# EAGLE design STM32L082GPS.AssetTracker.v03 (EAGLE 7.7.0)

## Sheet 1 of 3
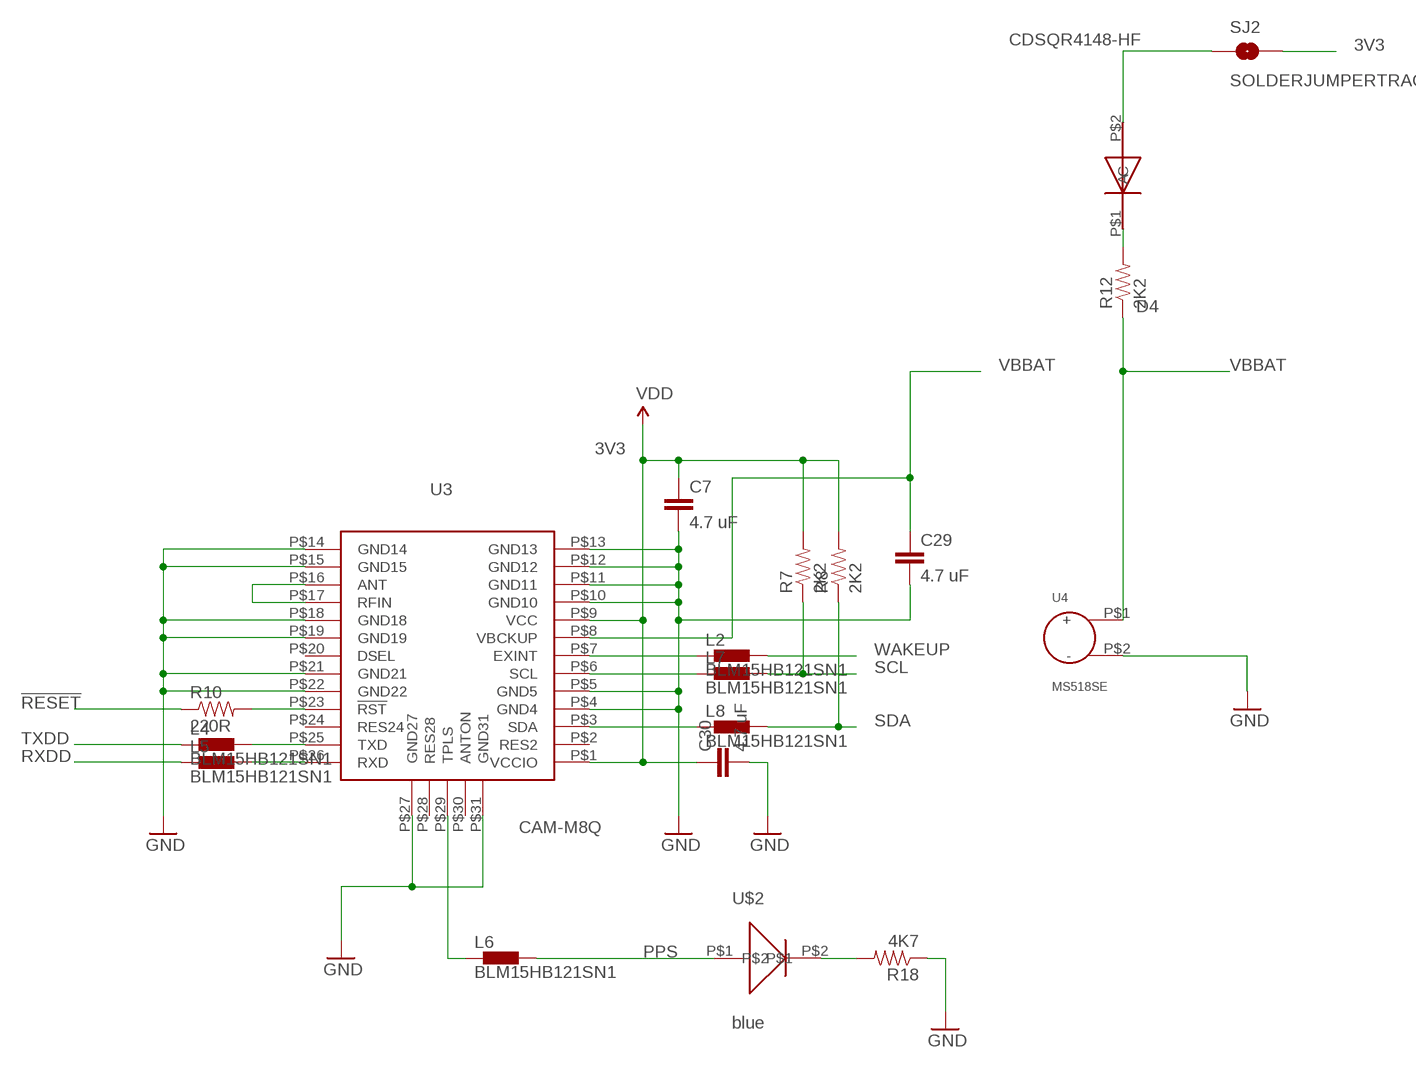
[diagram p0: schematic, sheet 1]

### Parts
C7  4.7 uF  0402CAP.KW  [0402-CAP]
C29  4.7 uF  0402CAP.KW  [0402-CAP]
C30  4.7 uF  0402CAP.KW  [0402-CAP]
D4  CDSQR4148-HF  [CDSQR4148-HF]
L2  BLM15HB121SN1  [0402]
L4  BLM15HB121SN1  [0402]
L5  BLM15HB121SN1  [0402]
L6  BLM15HB121SN1  [0402]
L7  BLM15HB121SN1  [0402]
L8  BLM15HB121SN1  [0402]
R7  2K2  0402RES.KW  [0402-RES]
R8  2K2  0402RES.KW  [0402-RES]
R10  220R  0402RES.KW  [0402-RES]
R12  2K2  0402RES.KW  [0402-RES]
R18  4K7  0402RES.KW  [0402-RES]
SJ2  SOLDERJUMPERTRACE  [SJ_2S-TRACE]
U3  CAM-M8Q  [CAM-M8Q]
U4  MS518SE  [MS518SE]
U$2  blue  0402LED  [0402LED]

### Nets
3V3: C7.1 C30.1 R7.2 R8.2 SJ2.2 U3.P$1(VCCIO) U3.P$9(VCC) ; supply symbol labelled VDD ; also sheet 2,3
!RESET: R10.1
GND: C7.2 C29.2 C30.2 R18.1 U3.P$4(GND4) U3.P$5(GND5) U3.P$10(GND10) U3.P$11(GND11) U3.P$12(GND12) U3.P$13(GND13) U3.P$14(GND14) U3.P$15(GND15) U3.P$18(GND18) U3.P$19(GND19) U3.P$21(GND21) U3.P$22(GND22) U3.P$27(GND27) U3.P$31(GND31) U4.P$2(-) ; also sheet 2,3
N$4: D4.P$2(A) SJ2.1
N$5: D4.P$1(C) R12.2
N$6: L2.1 U3.P$7(EXINT)
N$8: R18.2 U$2.P$2
N$10: L7.1 U3.P$6(SCL)
N$23: L8.1 U3.P$3(SDA)
N$43: L4.2 U3.P$25(TXD)
N$44: L5.2 U3.P$26(RXD)
N$45: U3.P$16(ANT) U3.P$17(RFIN)
N$46: R10.2 U3.P$23(!RST)
N$47: L6.1 U3.P$29(TPLS)
PPS: L6.2 U$2.P$1 ; also sheet 3
RXDD: L5.1 ; also sheet 3
SCL: L7.2 R7.1 ; also sheet 2,3
SDA: L8.2 R8.1 ; also sheet 2,3
TXDD: L4.1 ; also sheet 3
VBBAT: C29.1 R12.1 U3.P$8(VBCKUP) U4.P$1(+)
WAKEUP: L2.2 ; also sheet 3
Unconnected: U3.P$2(RES2) U3.P$20(DSEL) U3.P$24(RES24) U3.P$28(RES28) U3.P$30(ANTON)

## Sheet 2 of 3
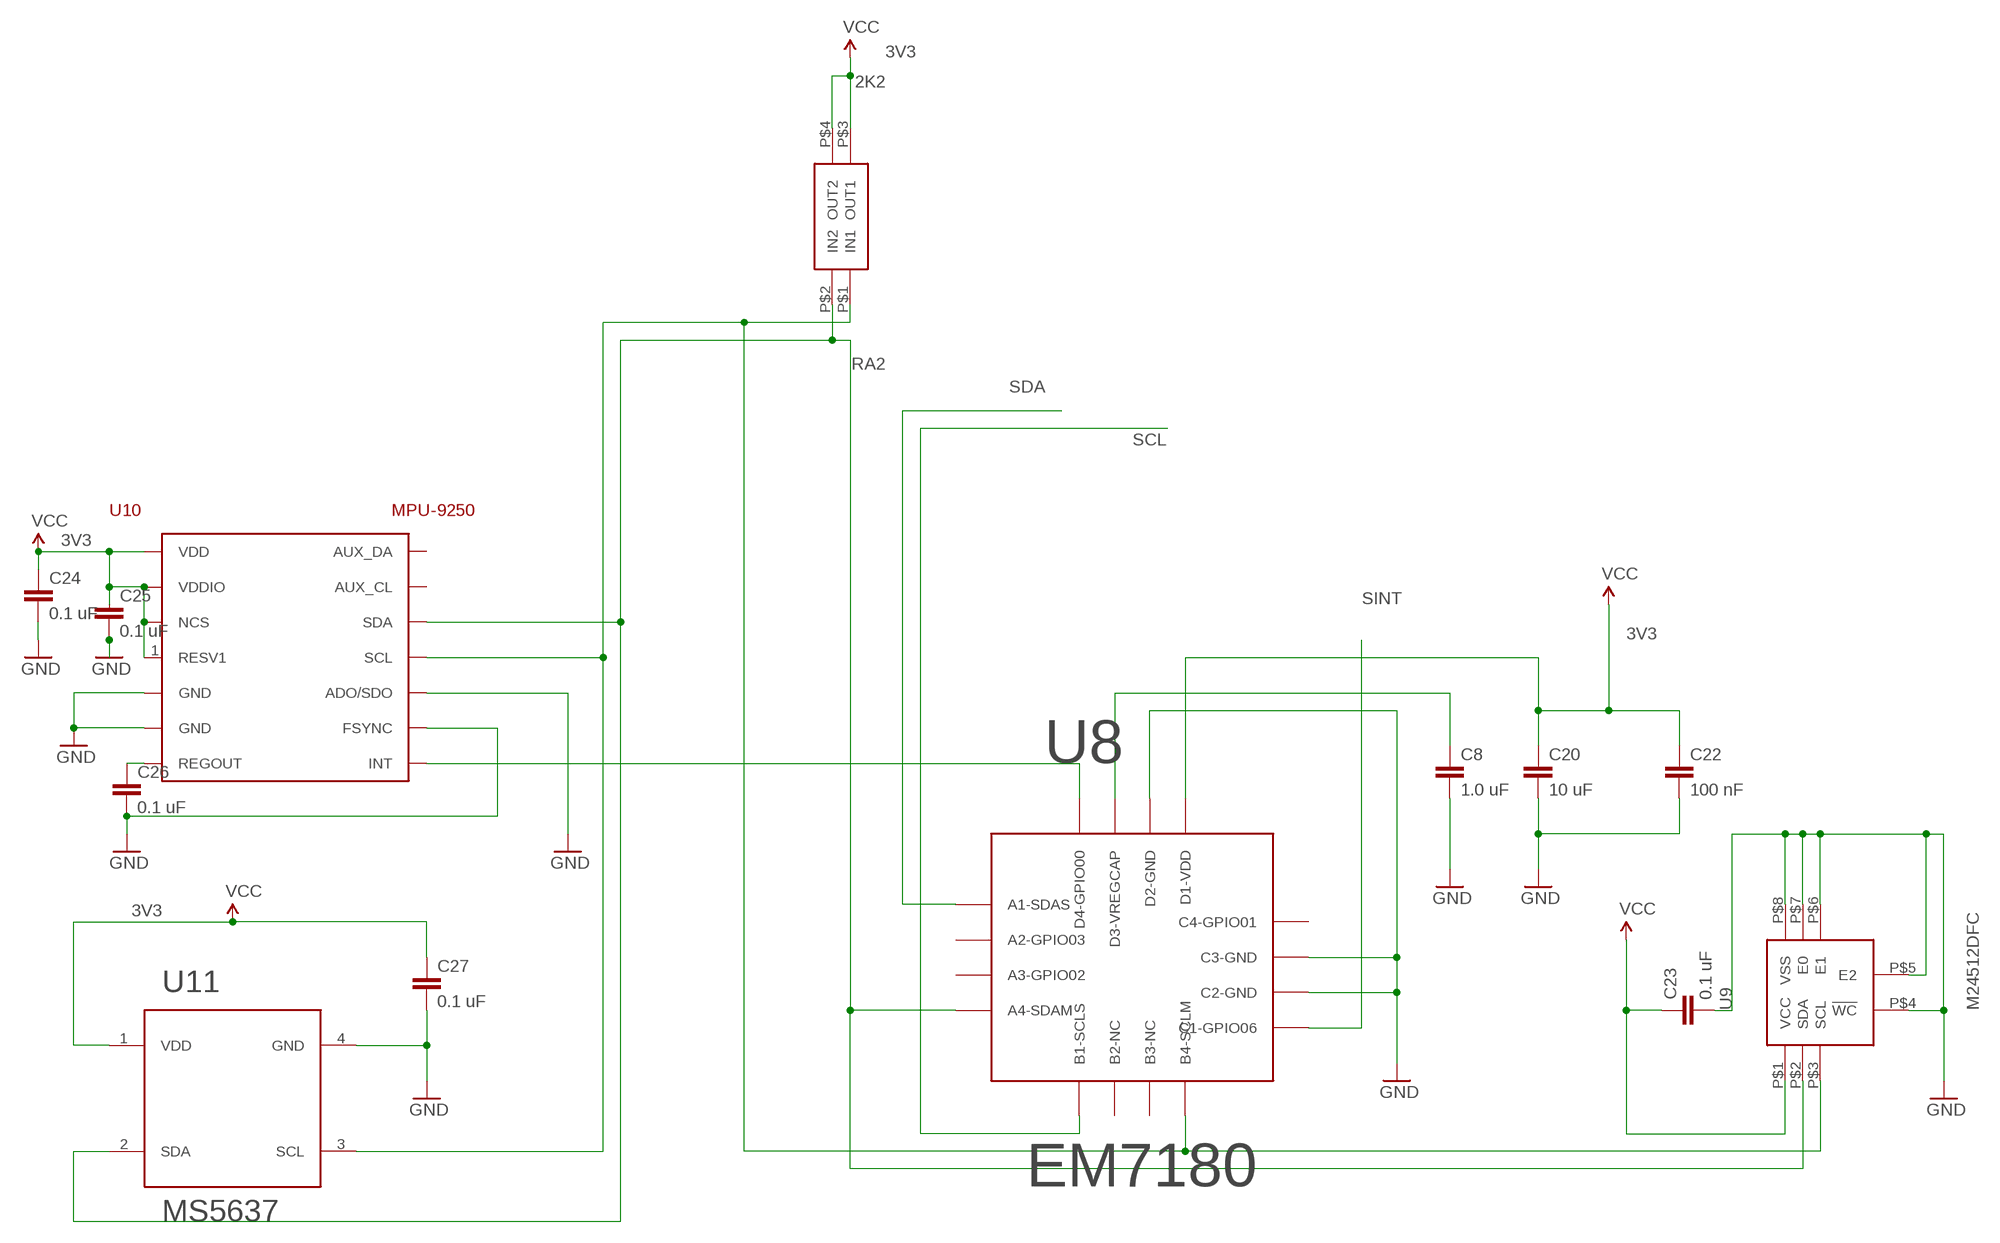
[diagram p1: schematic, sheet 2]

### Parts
C8  1.0 uF  CAP0402-CAP  [0402-CAP]
C20  10 uF  CAP0402-CAP  [0402-CAP]
C22  100 nF  CAP0402-CAP  [0402-CAP]
C23  0.1 uF  CAP0402-CAP  [0402-CAP]
C24  0.1 uF  CAP0402-CAP  [0402-CAP]
C25  0.1 uF  CAP0402-CAP  [0402-CAP]
C26  0.1 uF  CAP0402-CAP  [0402-CAP]
C27  0.1 uF  CAP0402-CAP  [0402-CAP]
RA2  2K2  EXB24V  [EXB24V]
U8  EM7180  [WL-CSP16]
U9  M24512DFC  [M24512DFC]
U10  MPU-9250  [MPU-9250]
U11  MS5637  [MS5637QFN-4]

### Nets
3V3: C20.1 C22.1 C23.1 C24.1 C25.1 C27.1 RA2.P$3(OUT1) RA2.P$4(OUT2) U8.P$13(D1-VDD) U9.P$1(VCC) U10.1(RESV1) U10.8(VDDIO) U10.13(VDD) U10.22(NCS) U11.1(VDD) ; supply symbol labelled VCC ; also sheet 1,3
GND: C8.2 C20.2 C22.2 C23.2 C24.2 C25.2 C26.2 C27.2 U8.P$10(C2-GND) U8.P$11(C3-GND) U8.P$14(D2-GND) U9.P$4(!WC) U9.P$5(E2) U9.P$6(E1) U9.P$7(E0) U9.P$8(VSS) U10.9(ADO/SDO) U10.11(FSYNC) U10.18(GND) U10.20(GND) U11.4(GND) ; also sheet 1,3
N$19: U8.P$16(D4-GPIO00) U10.12(INT)
N$26: C8.1 U8.P$15(D3-VREGCAP)
N$40: C26.1 U10.10(REGOUT)
SCL: U8.P$5(B1-SCLS) ; also sheet 1,3
SCL2: RA2.P$1(IN1) U8.P$8(B4-SCLM) U9.P$3(SCL) U10.23(SCL) U11.3(SCL)
SDA: U8.P$1(A1-SDAS) ; also sheet 1,3
SDA2: RA2.P$2(IN2) U8.P$4(A4-SDAM) U9.P$2(SDA) U10.24(SDA) U11.2(SDA)
SINT: U8.P$9(C1-GPIO06) ; also sheet 3
Unconnected: U8.P$2(A2-GPIO03) U8.P$3(A3-GPIO02) U8.P$6(B2-NC) U8.P$7(B3-NC) U8.P$12(C4-GPIO01) U10.7(AUX_CL) U10.21(AUX_DA)

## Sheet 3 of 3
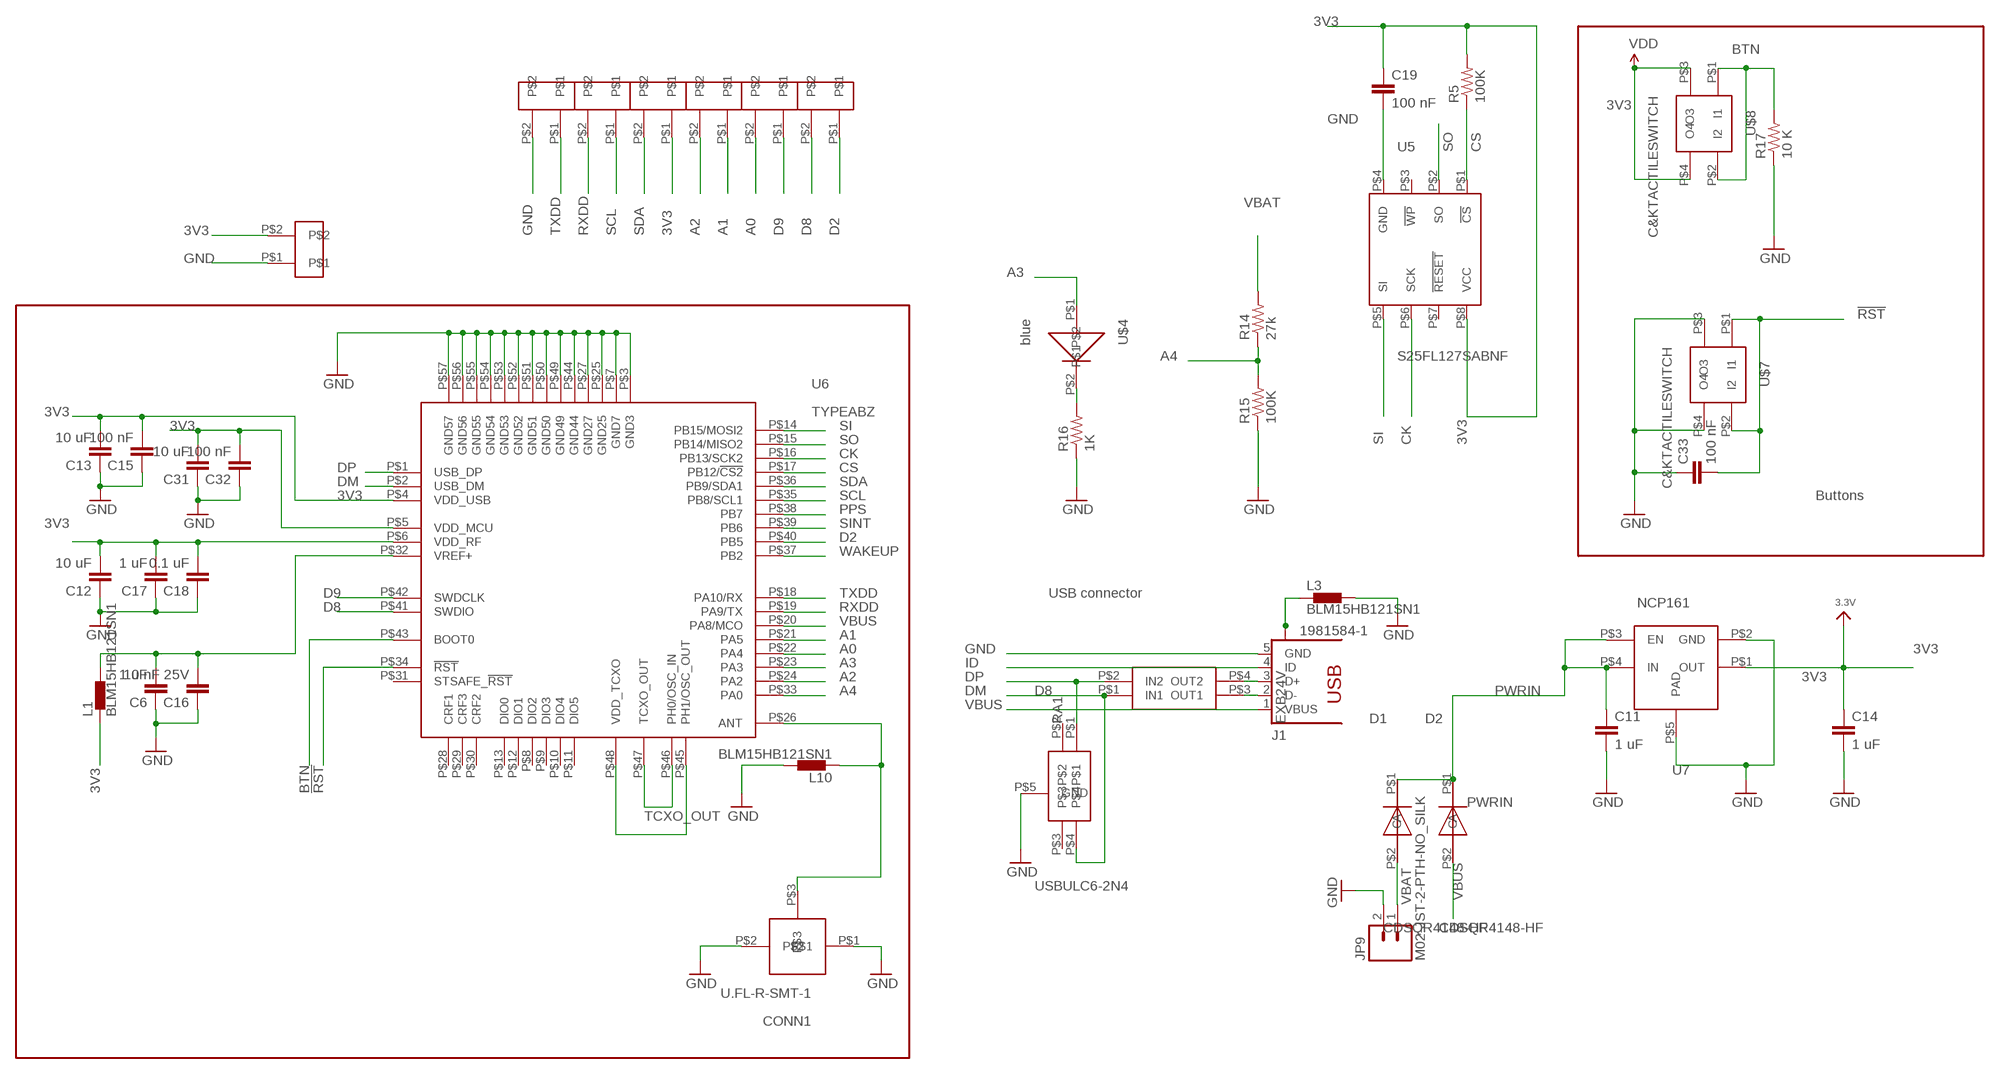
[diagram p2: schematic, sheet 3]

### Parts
C6  1 uF  0402CAP.KW  [0402-CAP]
C11  1 uF  CAP0402-CAP  [0402-CAP]
C12  10 uF  0402CAP.KW  [0402-CAP]
C13  10 uF  0402CAP.KW  [0402-CAP]
C14  1 uF  CAP0402-CAP  [0402-CAP]
C15  100 nF  0402CAP.KW  [0402-CAP]
C16  10 nF 25V  0402CAP.KW  [0402-CAP]
C17  1 uF  0402CAP.KW  [0402-CAP]
C18  0.1 uF  0402CAP.KW  [0402-CAP]
C19  100 nF  0402CAP.KW  [0402-CAP]
C31  10 uF  0402CAP.KW  [0402-CAP]
C32  100 nF  0402CAP.KW  [0402-CAP]
C33  100 nF  0402CAP.KW  [0402-CAP]
CONN1  U.FL-R-SMT-1  [U.FL-R-SMT-1]
D1  CDSQR4148-HF  [CDSQR4148-HF]
D2  CDSQR4148-HF  [CDSQR4148-HF]
D8  USBULC6-2N4  [USBULC6-2N4]
J1  1981584-1  [1981584-1]
JP9  M02-JST-2-PTH-NO_SILK  [JST-2-PTH-NS]
L1  BLM15HB121SN1  [0402]
L3  BLM15HB121SN1  [0402]
L10  BLM15HB121SN1  [0402]
R5  100K  0402RES.KW  [0402-RES]
R14  27k  0402RES.KW  [0402-RES]
R15  100K  0402RES.KW  [0402-RES]
R16  1K  0402RES.KW  [0402-RES]
R17  10 K  0402RES.KW  [0402-RES]
RA1  EXB24V  [EXB24V]
U5  S25FL127SABNF  [WSON-8]
U6  TYPEABZ  [TYPEABZ]
U7  NCP161  [NCP161]
U$4  blue  0402LED  [0402LED]
U$7  C&KTACTILESWITCH  [C&KTACTILESWITCH]
U$8  C&KTACTILESWITCH  [C&KTACTILESWITCH]
U$11  HN02  [HN02]
U$12  HN02  [HN02]
U$13  HN02  [HN02]
U$14  HN02  [HN02]
U$16  HN02  [HN02]
U$17  HN02  [HN02]
U$36  HN02  [HN02]

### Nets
3V3: C12.2 C13.2 C14.1 C15.2 C17.2 C18.2 C19.1 C31.2 C32.2 L1.1 R5.2 U5.P$8(VCC) U6.P$4(VDD_USB) U6.P$5(VDD_MCU) U6.P$6(VDD_RF) U7.P$1(OUT) U$8.P$3(O3) U$8.P$4(O4) U$13.P$1 U$36.P$2 ; supply symbol labelled VDD, 3.3V ; also sheet 1,2
!RST: C33.2 U6.P$34(!RST) U$7.P$1(I1) U$7.P$2(I2)
A0: U6.P$22(PA4) U$17.P$2
A1: U6.P$21(PA5) U$14.P$1
A2: U6.P$24(PA2) U$14.P$2
A3: U6.P$23(PA3) U$4.P$1
A4: R14.1 R15.2 U6.P$33(PA0)
AREF: C6.2 C16.2 L1.2 U6.P$32(VREF+)
BTN: R17.2 U6.P$43(BOOT0) U$8.P$1(I1) U$8.P$2(I2)
CK: U5.P$6(SCK) U6.P$16(PB13/SCK2)
CS: R5.1 U5.P$1(!CS) U6.P$17(PB12/!CS2)
D2: U6.P$40(PB5) U$16.P$1
D8: U6.P$41(SWDIO) U$16.P$2
D9: U6.P$42(SWDCLK) U$17.P$1
DM: D8.P$4 RA1.P$1(IN1) U6.P$2(USB_DM)
DP: D8.P$1 RA1.P$2(IN2) U6.P$1(USB_DP)
GND: C6.1 C11.2 C12.1 C13.1 C14.2 C15.1 C16.1 C17.1 C18.1 C19.2 C31.1 C32.1 C33.1 CONN1.P$1 CONN1.P$2 D8.P$5(GND) J1.5(GND) JP9.2 L3.2 L10.2 R15.1 R16.1 R17.1 U5.P$4(GND) U6.P$3(GND3) U6.P$7(GND7) U6.P$25(GND25) U6.P$27(GND27) U6.P$44(GND44) U6.P$49(GND49) U6.P$50(GND50) U6.P$51(GND51) U6.P$52(GND52) U6.P$53(GND53) U6.P$54(GND54) U6.P$55(GND55) U6.P$56(GND56) U6.P$57(GND57) U7.P$2(GND) U7.P$5(PAD) U$7.P$3(O3) U$7.P$4(O4) U$11.P$2 U$36.P$1 ; also sheet 1,2
ID: J1.4(ID)
N$7: U6.P$45(PH1/OSC_OUT) U6.P$48(VDD_TCXO)
N$11: R16.2 U$4.P$2
N$31: J1.3(D+) RA1.P$4(OUT2)
N$32: CONN1.P$3 L10.1 U6.P$26(ANT)
N$33: J1.2(D-) RA1.P$3(OUT1)
PPS: U6.P$38(PB7) ; also sheet 1
PWRIN: C11.1 D1.P$1(C) D2.P$1(C) U7.P$3(EN) U7.P$4(IN)
RXDD: U6.P$19(PA9/TX) U$12.P$2 ; also sheet 1
SCL: U6.P$35(PB8/SCL1) U$12.P$1 ; also sheet 1,2
SDA: U6.P$36(PB9/SDA1) U$13.P$2 ; also sheet 1,2
SI: U5.P$5(SI) U6.P$14(PB15/MOSI2)
SINT: U6.P$39(PB6) ; also sheet 2
SO: U5.P$2(SO) U6.P$15(PB14/MISO2)
TCXO_OUT: U6.P$46(PH0/OSC_IN) U6.P$47(TCXO_OUT)
TXDD: U6.P$18(PA10/RX) U$11.P$1 ; also sheet 1
USB_SHIELD1: J1.S1 J1.S2 J1.S3 J1.S4 L3.1
VBAT: D1.P$2(A) JP9.1 R14.2
VBUS: D2.P$2(A) J1.1(VBUS) U6.P$20(PA8/MCO)
WAKEUP: U6.P$37(PB2) ; also sheet 1
Unconnected: D8.P$2 D8.P$3 U5.P$3(!WP) U5.P$7(!RESET) U6.P$8(DIO2) U6.P$9(DIO3) U6.P$10(DIO4) U6.P$11(DIO5) U6.P$12(DIO1) U6.P$13(DIO0) U6.P$28(CRF1) U6.P$29(CRF3) U6.P$30(CRF2) U6.P$31(STSAFE_!RST)

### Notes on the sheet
- Buttons
- USB connector

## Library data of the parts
C6 C7 C12 C13 C15-C19 C29-C33 = SparkFun-Capacitors:0402CAP.KW
C8 C11 C14 C20 C22-C27 = SparkFun-Capacitors:CAP: Capacitor
CONN1 = Kris:U.FL-R-SMT-1: U.FL-R-SMT-1
D1 D2 D4 = Kris:CDSQR4148-HF: ComChip's CDSQR4148-HF high speed 150 mA Io diode
D8 = Kris:USBULC6-2N4: ST TVS diode ESD Protection USBULC6-2N4
J1 = con-usb:1981584-1: Receptacle, micro-USB, type A/B Tyco Electronics; MF: Hirose; MPN: ZX62-AB-5PA(11)
JP9 = SparkFun-Connectors:M02: Standard 2-pin 0.1" header. Use with
L1-L8 L10 = inductors:BLM15H: EMIFIL (R) Chip Ferrite Bead for GHz Noise
R5 R7 R8 R10 R12 R14-R18 = SparkFun-Resistors:0402RES.KW
RA1 RA2 = Kris:EXB24V: Panasonic EXB24 22 Ohm series resistor pair
SJ2 = SparkFun-Passives:SOLDERJUMPER: Solder Jumper
U3 = ubloxLib:CAM-M8Q: CAM-M8Q GPS/GNSS Module https://www.u-blox.com/sites/default/files/CAM-M8_HardwareIntegrationManual_%28UBX-14000014%29.pdf
U4 = Kris:MS518SE: S518SE 3 V rechargable Li battery
U5 = Kris:S25FL127SABNF: S225FL127SABNF1101 128 Mbit Spansion flash in WSON-8 package
U6 = Kris:TYPEABZ: CMWX1ZZABZ-078
U7 = Kris:NCP161: NCP161 3V3 LDO voltage regulator
U8 = SparkFun-DigitalIC:EM7180: WL-CSP19 package for the EM7180 SENtral sensor fusion hub
U9 = Kris:M24512DFC: ST's M24512DFC6 512 Mbit EEPROM
U10 = SparkFun-Sensors:MPU-9250: The MPU-9250 is a 9-axis motion sensor that contains an accelerometer/gyro sensor (MPU-6500) combined with a magnetometer (AK8963).
U11 = SparkFun-DiscreteSemi:MS5637: MS5637 I2C pressure sensor in QFN-4 package by Measurement Specialties
U$2 U$4 = Kris:0402LED: 0402led
U$7 U$8 = Kris:C&KTACTILESWITCH: C&K Tactile Switch 611-PTS810SJS250SMTR
U$11-U$14 U$16 U$17 U$36 = Kris:HN02: 0.1 inch header

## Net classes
1 USB: width 0.254 mm, drill 0.33 mm, clearance 0.159 mm
2 Top GND Pour: clearance 0.762 mm to class 1

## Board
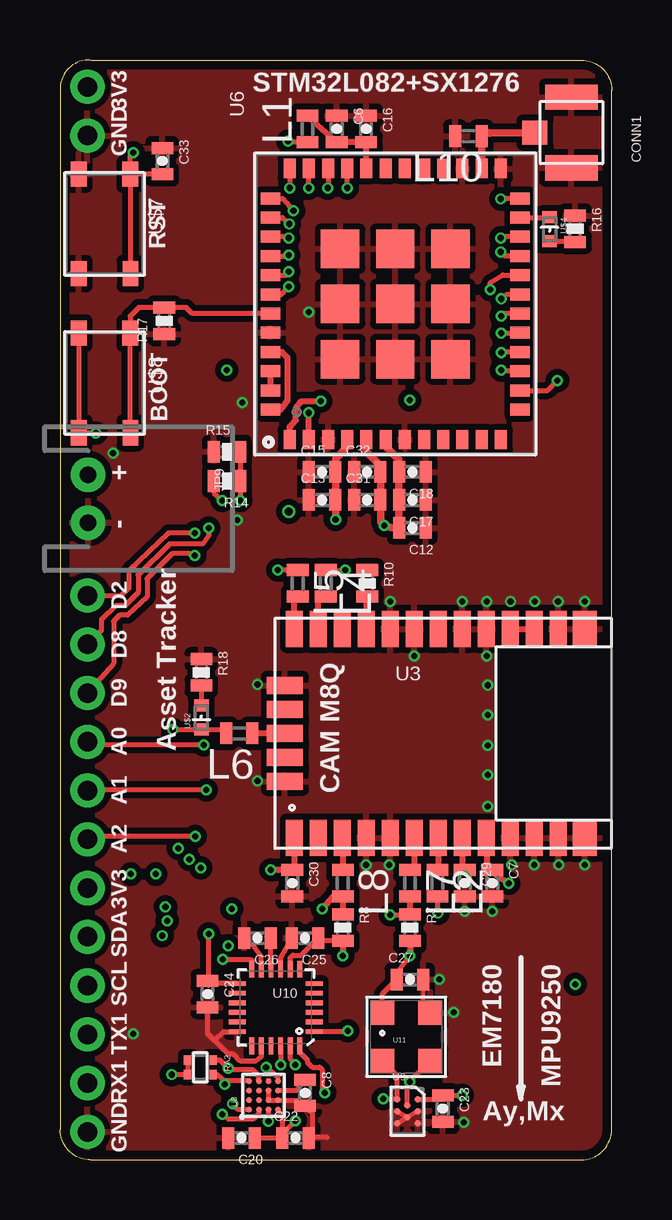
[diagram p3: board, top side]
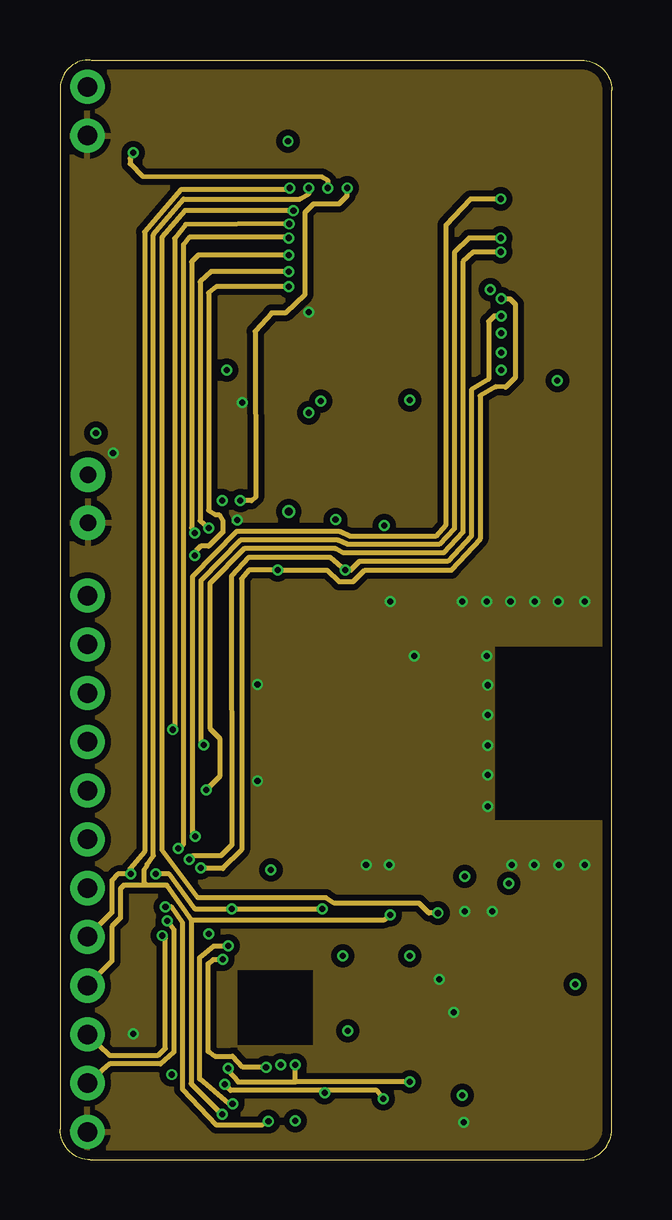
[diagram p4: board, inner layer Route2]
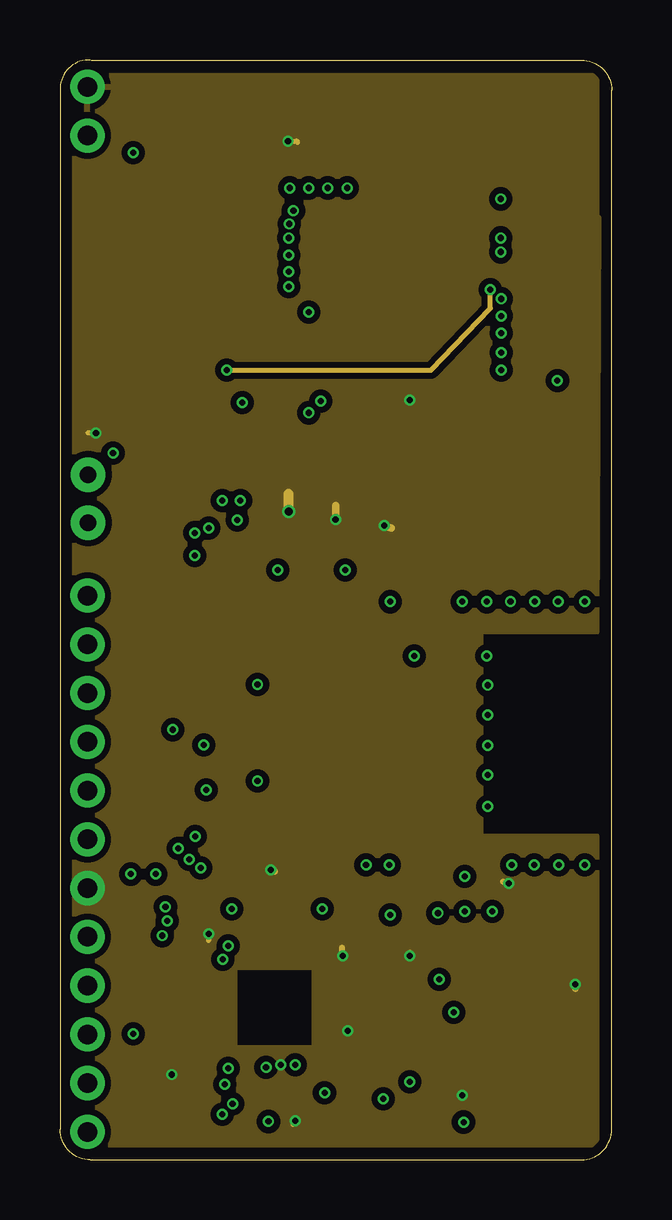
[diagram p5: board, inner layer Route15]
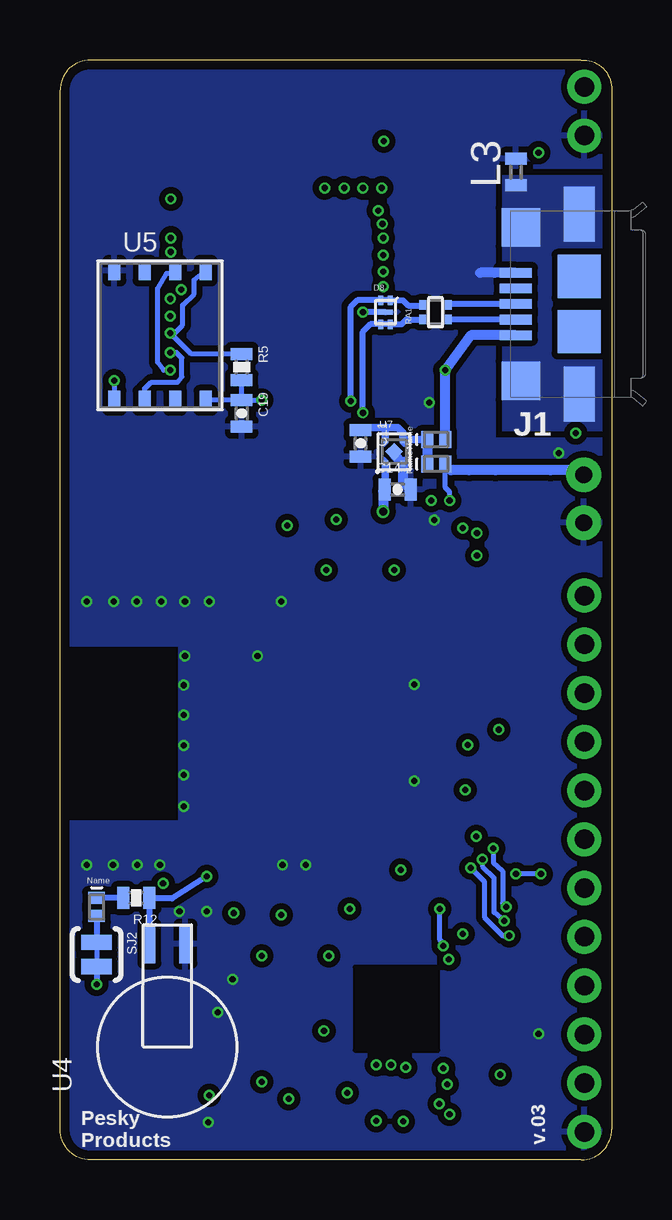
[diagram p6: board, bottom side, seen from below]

Size 22.99 x 45.85 mm. Coordinates in mm from the lower left corner, seen from the top.
Outline: 1.27,45.85 arc90 0,44.7 0,1.27 arc90 1.27,0 21.72,0 arc90 22.99,1.27 22.99,44.58 arc90 21.72,45.85 1.29,45.85
Copper layers (1*2*15*16): Top 0.035559375mm / dielectric 0.17018125mm / Route2 0.01778125mm / dielectric 47mil / Route15 0.01778125mm / dielectric 0.17018125mm / Bottom 0.035559375mm
Design rules "OSHPark-4layer *": minimum track width 5mil, minimum drill 10mil, track to track 5mil, track to pad 5mil, pad to pad 5mil, via to via 5mil, smd to smd 5mil, copper to edge 15mil, drill to drill 6mil, minimum pad ring 4mil, minimum via ring 4mil, stop-mask expansion 4mil, vias tented up to drill 20mil, thermal gap 10mil

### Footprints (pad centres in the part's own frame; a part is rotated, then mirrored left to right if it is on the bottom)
0402-CAP = smd 0.5 x 0.9: 1 -0.55,0; 2 0.55,0
U.FL-R-SMT-1 = smd 1.05 x 2.2: P$1 -1.475,0; P$2 1.475,0 | smd 1 x 1.05: P$3 0,-1.525
CDSQR4148-HF = smd 0.7 x 0.5: P$1 0,0.375; P$2 0,-0.375
USBULC6-2N4 = smd 0.2 x 0.4: P$1 0.2,0.5; P$2 -0.2,0.5; P$3 -0.2,-0.5; P$4 0.2,-0.5 | smd 0.6 x 0.2: P$5 0,0
1981584-1 = smd 0.4 x 1.35: 1 -1.3,4.1; 2 -0.65,4.1; 3 0,4.1; 4 0.65,4.1; 5 1.3,4.1 | smd 1.8 x 1.8: M1 -1.15,1.45; M2 1.15,1.45 | smd 2.3 x 1.3: S1 -3.75,1.45; S2 3.75,1.45 | smd 1.6 x 1.6: S3 -3.2,3.885; S4 3.2,3.885
JST-2-PTH-NS = drill 0.7 pad 1.448: 1 -1,0; 2 1,0
0402 = smd 0.5 x 0.9: 1 -0.55,0; 2 0.55,0
0402-RES = smd 0.5 x 0.9: 1 -0.55,0; 2 0.55,0
EXB24V = smd 0.4 x 0.36: P$1 -0.3,0.5; P$2 0.3,0.5; P$3 -0.3,-0.5; P$4 0.3,-0.5
SJ_2S-TRACE = smd 0.635 x 1.27: 1 -0.508,0; 2 0.508,0
CAM-M8Q = smd 0.7 x 1.5: P$1 0.8,0.45; P$2 1.8,0.45; P$3 2.8,0.45; P$4 3.8,0.45; P$5 4.8,0.45; P$6 5.8,0.45; P$7 6.8,0.45; P$8 7.8,0.45; P$9 8.8,0.45; P$10 9.8,0.45; P$11 10.8,0.45; P$12 11.8,0.45; P$15 11.8,9.15; P$16 10.8,9.15; P$17 9.8,9.15; P$18 8.8,9.15; P$19 7.8,9.15; P$20 6.8,9.15; P$21 5.8,9.15; P$22 4.8,9.15; P$23 3.8,9.15; P$24 2.8,9.15; P$25 1.8,9.15; P$26 0.8,9.15 | smd 1 x 1.5: P$13 12.9,0.45; P$14 12.9,9.15 | smd 1.5 x 0.7: P$27 0.4,6.8; P$28 0.4,5.8; P$29 0.4,4.8; P$30 0.4,3.8; P$31 0.4,2.8
MS518SE = smd 1.6 x 0.5: P$1 4.3,0.75; P$2 4.3,-0.75
WSON-8 = smd 0.5 x 0.8: P$1 1.905,2.7; P$2 0.635,2.7; P$3 -0.635,2.7; P$4 -1.905,2.7; P$5 -1.905,-2.7; P$6 -0.635,-2.7; P$7 0.635,-2.7; P$8 1.905,-2.7
TYPEABZ = smd 0.8 x 0.5: P$1 -5.65,4.4; P$2 -5.65,3.6; P$3 -5.65,2.8; P$4 -5.65,2; P$5 -5.65,1.2; P$6 -5.65,0.4; P$7 -5.65,-0.4; P$8 -5.65,-1.2; P$9 -5.65,-2; P$10 -5.65,-2.8; P$11 -5.65,-3.6; P$12 -5.65,-4.4; P$25 5.65,-4.4; P$26 5.65,-3.6; P$27 5.65,-2.8; P$28 5.65,-2; P$29 5.65,-1.2; P$30 5.65,-0.4; P$31 5.65,0.4; P$32 5.65,1.2; P$33 5.65,2; P$34 5.65,2.8; P$35 5.65,3.6; P$36 5.65,4.4 | smd 0.5 x 0.8: P$13 -4.4,-5.2; P$14 -3.6,-5.2; P$15 -2.8,-5.2; P$16 -2,-5.2; P$17 -1.2,-5.2; P$18 -0.4,-5.2; P$19 0.4,-5.2; P$20 1.2,-5.2; P$21 2,-5.2; P$22 2.8,-5.2; P$23 3.6,-5.2; P$24 4.4,-5.2; P$37 4.4,5.2; P$38 3.6,5.2; P$39 2.8,5.2; P$40 2,5.2; P$41 1.2,5.2; P$42 0.4,5.2; P$43 -0.4,5.2; P$44 -1.2,5.2; P$45 -2,5.2; P$46 -2.8,5.2; P$47 -3.6,5.2; P$48 -4.4,5.2 | smd 1.6 x 1.6: P$49 -2.3,2.3; P$50 0,2.3; P$51 2.3,2.3; P$52 -2.3,0; P$53 0,0; P$54 2.3,0; P$55 -2.3,-2.3; P$56 0,-2.3; P$57 2.3,-2.3
NCP161 = smd 0.24 x 0.24: P$1 -0.37,-0.48; P$2 0.37,-0.48; P$3 0.37,0.48; P$4 -0.37,0.48 | smd 0.52 x 0.52 rotated 45: P$5 0,0
WL-CSP16 = smd 0.24 x 0.24: P$1 -0.6,0.6; P$2 -0.2,0.6; P$3 0.2,0.6; P$4 0.6,0.6; P$5 -0.6,0.2; P$6 -0.2,0.2; P$7 0.2,0.2; P$8 0.6,0.2; P$9 -0.6,-0.2; P$10 -0.2,-0.2; P$11 0.2,-0.2; P$12 0.6,-0.2; P$13 -0.6,-0.6; P$14 -0.2,-0.6; P$15 0.2,-0.6; P$16 0.6,-0.6
M24512DFC = smd 0.27 x 0.27: P$1 0.433,0.5; P$2 -0.433,0.5; P$3 0,0.25; P$4 0.433,0; P$5 -0.433,0; P$6 0,-0.25; P$7 0.433,-0.5; P$8 -0.433,-0.5
MPU-9250 = smd 0.7 x 0.2: 1 -1.6,1; 2 -1.6,0.6; 3 -1.6,0.2; 4 -1.6,-0.2; 5 -1.6,-0.6; 6 -1.6,-1; 13 1.6,-1; 14 1.6,-0.6; 15 1.6,-0.2; 16 1.6,0.2; 17 1.6,0.6; 18 1.6,1 | smd 0.2 x 0.7: 7 -1,-1.6; 8 -0.6,-1.6; 9 -0.2,-1.6; 10 0.2,-1.6; 11 0.6,-1.6; 12 1,-1.6; 19 1,1.6; 20 0.6,1.6; 21 0.2,1.6; 22 -0.2,1.6; 23 -0.6,1.6; 24 -1,1.6
MS5637QFN-4 = smd 1 x 1: 1 -1,1; 2 -1,-1; 3 1,-1; 4 1,1
0402LED = smd 0.5 x 0.6: P$1 -0.5,0; P$2 0.5,0
C&KTACTILESWITCH = smd 1.05 x 0.65: P$1 -2.075,1.073; P$2 2.075,1.075; P$3 -2.075,-1.075; P$4 2.075,-1.075
HN02 = drill 0.813 pad 1.422: P$1 0,0; P$2 -2.032,0

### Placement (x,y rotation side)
C6  11.53,42.98 270 top
C7  18.01,11.53 270 top
C8  10.21,2.79 270 top
C11  10.46,29.87 270 bottom
C12  14.68,26.34 180 top
C13  10.92,27.51 0 top
C14  8.92,27.94 0 bottom
C15  10.92,28.68 0 top
C16  12.75,42.98 270 top
C17  14.68,27.51 180 top
C18  14.68,28.68 180 top
C19  15.42,31.11 270 bottom
C20  7.57,0.91 180 top
C22  9.8,0.91 0 top
C23  15.95,2.13 270 top
C24  6.15,6.91 270 top
C25  10.21,9.25 180 top
C26  8.23,9.25 180 top
C27  14.58,7.52 0 top
C29  16.87,11.53 270 top
C30  9.68,11.53 270 top
C31  12.8,27.51 0 top
C32  12.8,28.68 0 top
C33  4.27,41.63 270 top
CONN1  21.31,42.82 270 top
D1  7.32,29.01 90 bottom
D2  7.32,30.02 90 bottom
D4  21.46,10.54 0 bottom
D8  9.42,35.33 0 bottom
J1  -0.1,35.68 90 bottom
JP9  1.17,27.56 270 top
L1  10.31,42.98 90 top
L2  15.72,11.53 270 top
L3  3.99,41.17 90 bottom
L4  11.07,24.03 270 top
L5  9.91,24.03 270 top
L6  7.47,17.78 180 top
L7  14.58,11.53 270 top
L8  11.79,11.53 270 top
L10  17.02,42.67 180 top
R5  15.42,33.05 270 bottom
R7  14.58,9.68 270 top
R8  11.79,9.68 270 top
R10  12.8,24.03 270 top
R12  19.81,10.92 180 bottom
R14  6.96,28.3 180 top
R15  6.96,29.51 0 top
R16  21.46,38.81 270 top
R17  4.34,34.98 90 top
R18  5.89,20.32 270 top
RA1  7.34,35.33 90 bottom
RA2  5.84,3.86 270 top
SJ2  21.46,8.56 270 bottom
U3  8.97,12.98 0 top
U4  18.52,4.7 90 bottom
U5  18.82,34.37 0 bottom
U6  13.97,35.68 90 top
U7  9.07,29.51 0 bottom
U8  8.48,2.69 90 top
U9  14.48,2.03 0 top
U10  8.99,6.35 180 top
U11  14.43,5.13 0 top
U$2  5.89,18.44 90 top
U$4  20.4,38.79 270 top
U$7  1.85,39.01 270 top
U$8  1.85,32.38 270 top
U$11  1.14,3.2 90 top
U$12  1.14,7.26 90 top
U$13  1.14,11.33 90 top
U$14  1.14,15.39 90 top
U$16  1.14,23.52 90 top
U$17  1.14,19.46 90 top
U$36  1.14,42.7 270 top

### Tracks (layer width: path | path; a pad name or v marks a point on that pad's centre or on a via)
3V3  (via drill 0.25, 0.33)
  Top 0.203: U8.P$13 9.25,1.75 C22.1 | C22.1 9.2,0.97 v9.8,1.63 | U10.22 v9.2,3.96 | U11.1 13.43,6.92 C27.1 14.03,7.78 v14.58,8.51 | v16.76,2.69 16.81,2.68 C23.1 16.05,2.53 U9.P$1 | v4.65,3.56 RA2.P$4 RA2.P$3 | R8.2 10.96,9.13 C25.1 10.05,8.53 9.7,8.53 9.59,8.42 U10.8 | v6.2,9.42 6.2,7.26 C24.1 6.17,7.35 U10.13 | U10.1 11.95,5.35 v11.99,5.38 | C20.1 C22.1 | v1.5,30.3 1.19,30.31 U$8.P$4 U$8.P$3 | L1.1 9.59,42.43 v9.5,42.47
  Top 0.254: U3.P$9 17.79,12.4 C7.1 18.18,11.88 v18.69,11.53 | R7.2 14.59,8.75 v14.58,8.51 | R8.2 v11.79,8.51 | U3.P$1 9.77,12.09 C30.1 9.11,12.08 v8.79,12.09
  Top 0.305: U6.P$4 11.97,29.73 11.48,29.23 11.48,28.68 | 11.48,28.68 C15.2 | 11.48,28.68 11.48,27.52 C13.2 11.48,27.5 v11.48,26.7 | U6.P$6 13.57,29.74 14.12,29.18 C18.2 | C18.2 | C17.2 14.12,26.37 C12.2 13.78,26.36 v13.51,26.44 13.36,26.59 C31.2 | C18.2 C17.2 | C17.2 | U6.P$5 12.77,29.52 13.36,28.93 C32.2 | C32.2 | C32.2 C31.2 | C31.2
  Route15 0.203: v9.8,1.63 9.7,1.47 | v9.2,3.96 9.25,3.96 | v16.76,2.69 16.82,2.64 | v4.65,3.56 4.78,3.56 | v6.2,9.42 6.2,9.14 | v11.99,5.38 11.94,5.38 11.89,5.33 | v1.5,30.3 1.17,30.3 | v14.58,31.67 14.55,31.77 14.63,31.7 | v9.5,42.47 9.86,42.47 9.91,42.42
  Route15 0.254: 18.47,11.61 v18.69,11.53 | v14.58,8.51 14.58,8.64 | v11.79,8.51 11.76,8.84 | v8.79,12.09 8.97,12.01 8.91,12.06 8.91,12.09 8.87,12.14 | v21.46,7.32 21.46,7.14 21.49,7.11
  Route15 0.305: v11.48,26.7 11.48,27.28 | v13.51,26.44 13.79,26.34
  Route15 0.406: v9.53,27.03 9.53,27.76
  Bottom 0.203: C19.1 U5.P$8 | C19.1 v14.59,31.66 v14.58,31.67 | C19.1 R5.2
  Bottom 0.254: SJ2.2 v21.46,7.32
  Bottom 0.305: U7.P$1 9.44,28.4 C14.1 9.53,27.86
  Bottom 0.406: 9.53,27.86 v9.53,27.03
  pour Route15 (isolate 0.254, no thermals): 0.64,0.64 0.64,39.27 22.43,39.27 22.35,22.02 17.5,22.02 17.5,13.49 22.35,13.49 22.35,0.64 10.62,0.64 10.62,8.03 7.26,8.03 7.26,4.67 10.57,4.67 10.57,0.64
  pour Route15 (isolate 0.254): 0.64,39.27 0.64,45.19 22.35,45.19 22.35,39.27
!RST  (via drill 0.25)
  Top 0.203: C33.2 U$7.P$1 | U$7.P$1 U$7.P$2 | U6.P$34 11.17,40.66 v11.15,40.51 | U$7.P$1 2.92,41.83 v3.05,41.99
  Route2 0.203: v3.05,41.99 2.93,41.75 2.93,41.52 3.45,40.99 10.92,40.97 11.18,40.82 v11.15,40.51
A0  (via drill 0.25)
  Top 0.203: U6.P$22 18.41,38.48 v18.36,38.43 | v5.99,17.3 1.27,17.3 U$17.P$2
  Route2 0.203: v18.36,38.43 17.04,38.43 16.43,37.82 16.43,26.31 15.8,25.65 11.99,25.65 11.58,25.83 7.52,25.83 5.87,24.16 5.87,17.42 v5.99,17.3
A1  (via drill 0.25)
  Top 0.203: U6.P$21 18.53,37.68 v18.36,37.85 | v6.1,15.42 1.17,15.42 U$14.P$1
  Route2 0.203: v18.36,37.85 17.22,37.85 16.79,37.44 16.79,26.16 15.98,25.3 11.81,25.3 11.48,25.48 7.67,25.48 6.25,24.03 6.25,17.98 6.66,17.58 6.66,15.98 v6.1,15.42
A2  (via drill 0.25)
  Top 0.203: U6.P$24 18.39,40.08 v18.36,40.06 | v5.64,13.49 1.32,13.49 U$14.P$2
  Route2 0.203: v18.36,40.06 17.09,40.06 16.08,38.96 16.08,26.47 15.65,25.98 12.09,25.98 11.66,26.19 7.34,26.19 5.51,24.31 5.51,13.59 v5.64,13.49
A3
  Top 0.203: U6.P$23 20.34,39.28 U$4.P$1
A4  (via drill 0.25)
  Top 0.203: R15.2 R14.1 7.51,27.52 v7.52,27.48 | v11.96,40.51 U6.P$33
  Route2 0.203: v11.96,40.51 11.96,40.18 11.63,39.85 10.57,39.85 10.21,39.5 10.21,36.07 9.4,35.31 8.81,35.31 8.13,34.54 8.15,27.61 7.98,27.48 v7.52,27.48
AREF
  Top 0.254: U6.P$32 12.77,42.41 | C16.2 C6.2 L1.2
  Top 0.305: 12.77,42.41 C16.2
BTN
  Top 0.203: U6.P$43 5.52,35.28 5.26,35.53 4.35,35.53 | 4.35,35.53 R17.2 | U$8.P$2 U$8.P$1 2.92,35.18 3.28,35.53 4.35,35.53
CK  (via drill 0.25)
  Top 0.203: U6.P$16 18.41,33.68 v18.39,33.66
  Bottom 0.203: U5.P$6 19.46,32.16 19.18,32.41 18.09,32.41 17.91,32.64 17.91,33.43 18.14,33.66 v18.39,33.66
CS  (via drill 0.25)
  Top 0.203: v18.39,34.47 19.16,34.47 U6.P$17
  Bottom 0.203: 16.9,37.05 U5.P$1 17.4,36.69 17.4,36.09 17.88,35.64 17.88,34.8 18.21,34.47 v18.39,34.47 17.52,33.59 R5.1
D2  (via drill 0.25)
  Top 0.203: U6.P$40 9.43,37.68 v9.53,37.72 | v5.61,26.14 4.52,26.14 2.87,24.54 2.87,23.82 2.54,23.5 1.17,23.5 U$16.P$1
  Route2 0.203: v9.53,37.72 5.77,37.72 5.49,37.44 5.49,26.34 v5.61,26.14
D8  (via drill 0.25)
  Top 0.203: U6.P$41 9.42,36.88 v9.53,37.03 | v6.2,26.34 6.2,26.04 5.94,25.68 4.57,25.68 3.25,24.38 3.25,23.65 2.72,23.11 2.34,23.11 1.73,22.5 1.73,22.07 U$16.P$2
  Route2 0.203: v9.53,37.03 6.3,37.03 5.84,36.6 5.84,26.64 v6.2,26.34
D9  (via drill 0.25)
  Top 0.203: U6.P$42 9.23,36.08 v9.53,36.4 | v5.61,25.2 5.61,25.25 5.39,25.27 4.67,25.27 3.63,24.23 3.63,23.47 2.82,22.71 2.49,22.71 2.24,22.45 2.24,20.7 U$17.P$1
  Route2 0.203: v9.53,36.4 6.5,36.4 6.2,36.14 6.2,27.08 6.48,26.9 6.63,26.9 6.78,26.64 6.78,26.16 6.2,25.58 5.87,25.58 5.66,25.38 v5.61,25.2
DM  (via drill 0.25)
  Top 0.254: U6.P$2 10.37,31.17 v10.36,31.14
  Bottom 0.254: v10.36,31.14 10.36,34.52 10.05,34.83 D8.P$4 8.75,34.83 8.56,35.03 RA1.P$1
DP  (via drill 0.25)
  Top 0.254: U6.P$1 9.57,30.55 9.83,30.84 9.83,31.34 10.06,31.62 v10.87,31.62
  Bottom 0.254: v10.87,31.62 10.87,35.56 10.6,35.83 D8.P$1 8.7,35.83 8.48,35.61 7.86,35.61 RA1.P$2
GND  (via drill 0.25)
  Top 0.152: C27.2 15.13,6.43 U11.4
  Top 0.203: U8.P$11 U8.P$10 U8.P$14 9.96,2.49 C8.2 10.52,1.93 10.52,1.08 C22.2 10.35,0.94 11.12,0.94 | U10.11 8.39,8.47 8.08,8.89 C26.2 | U10.9 9.19,8.42 C25.2 | U10.18 7.37,5.32 6.8,5.32 6.45,4.98 | U9.P$5 U9.P$6 | U9.P$8 U9.P$6 | U9.P$4 U9.P$6 | U10.20 8.39,4.3 8.15,4.12 7.52,4.12 7.21,4.42 7.01,4.42 6.45,4.98 | 6.45,4.98 6.43,4.98 6.15,5.26 C24.2 | 10.36,0.84 10.36,0.86
  Top 0.254: C22.2 10.35,0.87 10.36,0.86 | v10.36,35.33 10.31,35.28
  Bottom 0.254: D8.P$5 v10.36,35.33
  Bottom 0.406: J1.5 4.88,36.98 5.49,36.98 | C14.2 8.7,28.27 U7.P$2 9.07,29.41 U7.P$5
  other vias: 20.75,23.27 21.87,23.27 17.78,21.01 16.76,23.27 18.82,12.29 19.76,12.29 20.78,12.29 21.87,12.29 14.76,21.01 13.77,23.27 13.72,12.29 12.75,12.29 8.23,19.81 8.23,15.8 17.83,19.79 17.83,18.54 17.83,17.27 17.83,16.05 17.83,14.73 18.01,10.36 16.41,6.15 15.8,7.52 16.81,1.57 3.05,5.26 7.39,26.67 17.78,23.27 18.77,23.27 16.87,10.36 19.79,23.27 7.59,31.57 2.21,29.46
  pour Top (isolate 0.254): 0,0 0,39.29 22.99,39.29 23.06,21.51 17.98,21.51 17.98,14.05 22.96,14.05 22.96,0 16,0 16,6.76 12.75,6.76 12.75,3.56 15.95,3.56 15.95,0 10.67,0 10.67,8.03 7.26,8.03 7.26,4.67 10.66,4.67 10.66,0
  pour Route2 (isolate 0.254): 0,0 0,39.27 22.99,39.27 23.04,21.51 17.98,21.51 17.98,14.05 23.04,14.05 22.99,0 10.67,0 10.67,8.03 7.26,8.03 7.26,4.67 10.62,4.67 10.62,0
  pour Route2 (isolate 0.254): 22.99,39.27 0,39.27 0,45.82 22.99,45.82
  pour Top (isolate 0.254): 0,39.27 0,45.82 22.99,45.82 22.99,39.27
  pour Bottom (isolate 0.254): 0,0 22.99,0 22.99,45.85 -0.03,45.85 -0.03,41.43 4.95,41.43 4.95,30 -0.13,30
N$1
  cutout Bottom: 7.29,8.03 10.69,8.03 10.69,4.57 7.24,4.57 7.24,8.03
N$2
  cutout Bottom (isolate 0.254): 23.04,21.39 18.11,21.39 18.11,14.17 23.04,14.17
N$4
  Bottom 0.254: D4.P$2 SJ2.1
N$5
  Bottom 0.254: R12.2 D4.P$1
N$6
  Top 0.254: U3.P$7 15.77,12.1 L2.1
N$7
  Top 0.254: U6.P$45 9.25,33.68 9.47,33.45 9.47,31.65 9.2,31.27 8.78,31.27 U6.P$48
N$8
  Top 0.203: R18.2 U$2.P$2
N$10
  Top 0.254: U3.P$6 14.77,12.27 L7.1
N$11
  Top 0.203: U$4.P$2 21.36,38.29 R16.2
N$19  (via drill 0.25)
  Top 0.203: U8.P$16 9.08,3.41 v8.59,3.86 | v6.78,8.36 7.93,8.36 7.99,8.32 U10.12
  Route2 0.203: v6.78,8.36 6.38,8.36 6.17,8.18 6.17,4.52 6.45,4.32 7.19,4.32 7.62,3.86 v8.59,3.86
N$23
  Top 0.254: U3.P$3 L8.1
N$26
  Top 0.203: U8.P$15 9.86,2.89 C8.1
N$31
  Bottom 0.254: J1.3 6.8,35.68 RA1.P$4
N$32
  Top 0.203: L10.1
  Top 0.305: U6.P$26 L10.1 | CONN1.P$3 17.9,42.8 arc90 L10.1
N$33
  Bottom 0.254: J1.2 5.49,35.03 RA1.P$3
N$40
  Top 0.203: U10.10 8.79,9.05 C26.1
N$43
  Top 0.254: U3.P$25 10.77,23.4 10.84,23.42 L4.2
N$44
  Top 0.254: U3.P$26 9.77,23.41 9.78,23.48 L5.2
N$45
  Top 0.254: U3.P$17 U3.P$16
N$46
  Top 0.254: U3.P$23 12.79,23.57 R10.2
N$47
  Top 0.254: U3.P$29 8.25,17.78 L6.1
PPS  (via drill 0.25)
  Top 0.203: U6.P$38 9.26,39.28 v9.55,39.01 | v4.7,17.93 U$2.P$1 6.76,17.94 L6.2
  Route2 0.203: v9.55,39.01 5.23,38.99 4.78,38.41 4.78,18.06 v4.7,17.93
PWRIN
  Bottom 0.305: D2.P$1 8.67,30.02 U7.P$3 8.7,30.31 8.91,30.52 9.45,30.52 | U7.P$4 9.44,30.51 9.45,30.52 | 9.45,30.52 10.36,30.52 C11.1
  Bottom 0.406: D2.P$1 D1.P$1
RXDD  (via drill 0.25)
  Top 0.203: v9.07,24.59 9.41,24.58 L5.1 | U6.P$19 18.6,36.08 v18.39,35.89
  Route2 0.203: U$12.P$2 2.08,4.34 4.06,4.34 4.39,4.65 4.39,9.25 v4.27,9.35 | v18.39,35.89 18.75,35.89 18.97,35.66 18.97,32.61 18.57,32.21 18.16,32.23 17.5,31.85 17.5,25.88 16.31,24.59 12.7,24.59 12.22,24.11 11.63,24.11 11.12,24.59 v9.07,24.59 7.87,24.59 7.57,24.23 7.57,12.93 6.78,12.14 5.89,12.14 v5.87,12.17
  Bottom 0.203: v5.87,12.17 5.31,11.61 5.31,10.11 4.55,9.35 v4.27,9.35 4.24,9.35
SCL  (via drill 0.25)
  Top 0.203: U8.P$5 8.28,1.93 8.05,1.7 7.01,1.7 v6.76,1.91 | v13.77,10.21 14.56,10.21 R7.1 | v10.36,40.51 U6.P$35
  Top 0.254: L7.2 R7.1
  Route2 0.203: 5.46,10.01 4.46,11.44 3.61,11.44 | 5.46,10.01 5.46,3.17 6.68,1.96 v6.76,1.91 | 5.46,10.01 13.51,10.01 v13.77,10.21 | 3.61,11.44 3.49,11.56 3.49,12.06 3.63,12.28 3.63,12.32 3.89,12.68 3.89,38.56 5.16,40.06 10.01,40.06 10.36,40.26 v10.36,40.51 | 3.61,11.44 2.65,11.44 2.52,11.3 2.52,10.08 2.16,9.73 2.16,8.28 U$12.P$1
SCL2  (via drill 0.25)
  Top 0.203: U8.P$8 8.28,3.5 8.03,3.76 7.06,3.76 v7.01,3.81 6.66,4.16 RA2.P$1 | U9.P$3 14.48,3.18 | 14.48,3.18 U11.3 | 14.48,3.18 14.55,3.18 v14.58,3.25 | v9.8,3.96 9.6,4.22 9.6,4.71 U10.23
  Route2 0.203: v14.58,3.25 9.8,3.25 | 9.8,3.25 v9.8,3.96 | v7.01,3.81 7.01,3.71 7.42,3.25 9.8,3.25
SDA  (via drill 0.25)
  Top 0.203: U8.P$1 7.43,2.09 v7.19,2.34 | U6.P$36 9.57,40.47 v9.58,40.51
  Top 0.254: R8.1 L8.2 11.39,10.98 v10.92,10.46
  Route2 0.203: 10.77,10.49 v10.92,10.46 v7.16,10.46 5.61,10.46 4.55,11.91 v3.99,11.91 | v7.19,2.34 7.04,2.34 5.82,3.38 5.82,8.43 6.4,8.91 v7.01,8.91 | U$13.P$2 2.16,10.31 2.16,11.66 2.41,11.91 v2.95,11.91 2.92,12.14 3.53,12.85 3.53,38.68 5.03,40.44 9.45,40.44 v9.58,40.51
  Bottom 0.203: v7.01,8.91 6.96,8.97 7.16,9.17 v7.16,10.46 | v2.95,11.91 v3.99,11.91
SDA2  (via drill 0.25)
  Top 0.203: U8.P$4 6.86,3.29 | 13.24,3.96 U11.2 14.05,3.51 U9.P$2 14.04,2.54 v13.46,2.54 | 6.86,3.29 6.86,3.26 v6.86,3.15 | RA2.P$2 6.55,3.56 6.86,3.29 | U10.24 9.99,4.49 10.31,4.17 10.31,4.06 10.52,3.86 10.82,3.86 10.92,3.76 10.92,2.9 v11.02,2.79
  Route2 0.203: v13.46,2.54 13.21,2.9 11.02,2.9 | 11.02,2.9 7.11,2.9 v6.86,3.15 | v11.02,2.79 11.02,2.9
SI  (via drill 0.25)
  Top 0.203: U6.P$14 20.32,32.08 v20.73,32.49
  Bottom 0.203: v20.73,32.49 U5.P$5
SINT  (via drill 0.25)
  Top 0.203: U8.P$9 v8.68,1.6 v8.69,1.6 | v9.53,38.43 9.38,38.48 U6.P$39
  Route2 0.203: v8.69,1.6 8.64,1.6 8.41,1.45 6.53,1.45 5.11,2.95 5.11,9.88 4.65,10.54 v4.39,10.54 | v4.93,12.98 5.16,13.16 5.16,38.15 5.41,38.48 9.35,38.48 v9.53,38.43
  Bottom 0.203: 4.52,10.62 v4.39,10.54 4.55,10.69 4.55,12.04 4.93,12.39 v4.93,12.98
SO  (via drill 0.25)
  Top 0.203: U6.P$15 18.41,32.88 v18.39,32.92
  Bottom 0.203: v18.39,32.92 18.67,32.92 18.92,33.25 18.92,36.32 18.54,36.96 18.19,36.96 U5.P$2
TCXO_OUT
  Top 0.254: U6.P$46 U6.P$47
TXDD  (via drill 0.25)
  Top 0.203: v11.89,24.59 11.2,24.54 L4.1 | U6.P$18 18.49,35.28 v18.39,35.18
  Route2 0.203: v4.47,9.96 4.75,9.6 4.75,4.5 4.18,4 2.07,4 U$11.P$1 | v18.39,35.18 18.09,35.18 17.86,34.95 17.86,32.54 17.14,32.11 17.14,26.01 16.15,24.94 12.47,24.94 12.12,24.59 v11.89,24.59 11.25,25.12 7.87,25.12 7.14,24.33 7.16,13.13 6.71,12.68 5.54,12.68 v5.39,12.52
  Bottom 0.203: v4.47,9.96 4.9,10.31 4.9,11.76 5.39,12.24 v5.39,12.52
USB_SHIELD1
  pour Bottom (isolate 0.254, rank 3, no thermals): 0,41.17 4.7,41.17 4.7,30.25 0,30.25
VBAT  (via drill 0.25)
  Top 0.203: R14.2 6.41,27.8 v6.76,27.48
  Bottom 0.203: 5.99,28.8 5.94,28.75 | v6.76,27.48 6.76,27.84 6.93,28.02 D1.P$2
  Bottom 0.254: 2.54,28.75 2.96,28.75 | 4.9,28.7 4.85,28.75
  Bottom 0.406: D1.P$2 6.88,28.85 6.71,28.75 5.94,28.75 4.85,28.75 2.54,28.75 1.58,28.75 JP9.1
VBBAT  (via drill 0.25)
  Top 0.254: U3.P$8 16.77,12.18 C29.1 v16.87,11.81
  Bottom 0.254: v16.87,11.81 18.31,10.9 19.24,10.9 R12.1 19.26,9.16 U4.P$1
VBUS  (via drill 0.25)
  Top 0.203: v17.93,36.27 17.93,36.58 18.44,36.88 U6.P$20
  Route15 0.203: v6.94,32.92 15.47,32.92 17.93,35.48 v17.93,36.27
  Bottom 0.406: D2.P$2 6.94,30.96 v6.94,32.92 5.87,34.38 J1.1
WAKEUP  (via drill 0.25)
  Top 0.203: L2.2 15.72,10.31 v15.75,10.29 | U6.P$37 9.28,40.08 v9.73,39.57
  Route2 0.203: v15.75,10.29 15.37,10.29 14.96,10.69 11.43,10.69 11.07,10.92 5.74,10.92 4.24,12.93 4.24,38.46 5.21,39.57 v9.73,39.57

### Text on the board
tPlace: STM32L082+SX1276 | 3V3 | GND | RST | BOOT | + | - | Asset Tracker | D2 | D8 | D9 | A0 | A1 | CAM M8Q | A2 | 3V3 | SDA | EM7180 | MPU9250 | SCL | TX1 | RX1 | Ay,Mx | GND
bPlace: v.03 | Pesky / Products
